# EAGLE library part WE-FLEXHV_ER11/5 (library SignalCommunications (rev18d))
WE-FLEX HV Flexible Transformer for DC/DC Converter Characteristics Transformer with 6 identical windings 4 sizes with 5 different lengths of air gap each Isolation voltage up to 1.5 kVAC Low leakage inductance Operating temperature: –40 ºC to +125 ºC By using different circuits more than 375 transformer solutions and about 125 choke solutions possible. Consequently, quick prototyping possibilities EFD size parts provide Basic insulation for a working voltage of 250VRMS when they are connteced approbiate Applications Flyback converters Forward converters Push-pull converters Step-up/step-down converters SEPIC Details see: http://katalog.we-online.de/en/pbs/WE-FLEXHV/749196308?m Created by Yingchun Shan 2017 (C) Wurth Elektronik
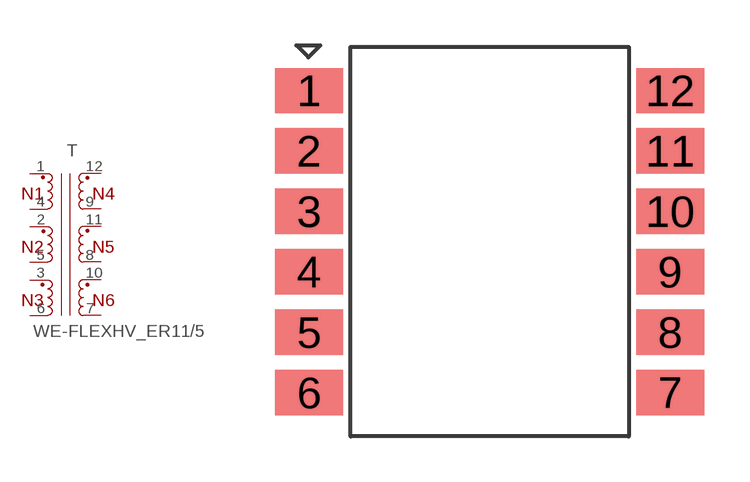
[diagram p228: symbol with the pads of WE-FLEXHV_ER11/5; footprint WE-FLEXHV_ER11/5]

Designator prefix T

## WE-FLEXHV_ER11/5_749196108 (WE-NUMBER: 749196108/224,6uH), WE-FLEXHV_ER11/5_749196118 (WE-NUMBER: 749196118/27,4uH), WE-FLEXHV_ER11/5_749196128 (WE-NUMBER: 749196128/14,7uH), WE-FLEXHV_ER11/5_749196138 (WE-NUMBER: 749196138/10,9uH), WE-FLEXHV_ER11/5_749196148 (WE-NUMBER: 749196148/8,5uH)  [WE-FLEXHV_ER11/5]
1  1  pas
2  2  pas
3  3  pas
4  4  pas
5  5  pas
6  6  pas
7  7  pas
8  8  pas
9  9  pas
10  10  pas
11  11  pas
12  12  pas

## Footprint WE-FLEXHV_ER11/5 (pad centres in mm)
smd 2.25 x 1.5: 1 -5.975,5; 2 -5.975,3; 3 -5.975,1; 4 -5.975,-1; 5 -5.975,-3; 6 -5.975,-5; 7 5.975,-5; 8 5.975,-3; 9 5.975,-1; 10 5.975,1; 11 5.975,3; 12 5.975,5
